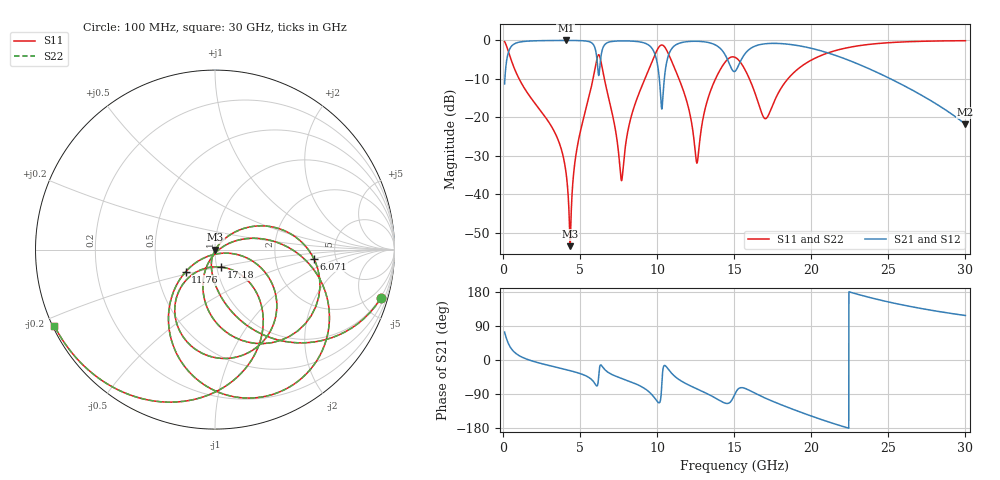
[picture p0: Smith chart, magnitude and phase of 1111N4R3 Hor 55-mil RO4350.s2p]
# GHz S MA R 50
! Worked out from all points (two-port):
!   3201 points, 100 MHz to 30 GHz, reference 50 ohm
!   highest |S21| = -0.02 dB at 4.071 GHz (marker M1); lowest = -21.8 dB at 30 GHz (marker M2)
!   |S21| within 3 dB of the highest: 352.9 MHz to 6.027 GHz (5.674 GHz wide, 178 % of centre); 15.79 GHz to 20.89 GHz (5.094 GHz wide, 27.8 % of centre)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
!   lowest |S11| = -53.5 dB at 4.351 GHz (marker M3), VSWR 1.00, Z = 50.2 - j0.11 ohm
!   |S11| at or under -10 dB: 1.04 GHz to 5.837 GHz (4.797 GHz wide, 140 % of centre); 6.574 GHz to 9.204 GHz (2.63 GHz wide, 33.3 % of centre); 15.98 GHz to 18.48 GHz (2.499 GHz wide, 14.5 % of centre)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
!   |S22| runs from -53.5 to -0.1 dB; largest |S21 - S12| = 0
!   S11 on the Smith chart (normalised r, x): 100 MHz: 0.93, -6.81; 6.071 GHz: 3.40, -0.49; 11.76 GHz: 0.70, -0.18; 17.18 GHz: 1.05, -0.21; 30 GHz: 0.00, -0.23
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0.1  0.9623 -16.4  0.2716 73.6  0.2716 73.6  0.9623 -16.4
1.015688  0.3233 -77.7  0.9456 12.2  0.9456 12.2  0.3233 -77.7
4.071094  0.01998 -110.4  0.9977 -25.2  0.9977 -25.2  0.01998 -110.4
4.351406  0.002103 -31.5  0.9974 -28.1  0.9974 -28.1  0.002103 -31.5
5.089563  0.07556 48.7  0.991 -37.1  0.991 -37.1  0.07556 48.7
6.070656  0.5528 -5.2  0.6197 -68.4  0.6197 -68.4  0.5528 -5.2
6.313594  0.5785 -64.9  0.5312 -13.3  0.5312 -13.3  0.5785 -64.9
6.60325  0.2959 -100.7  0.8825 -25.4  0.8825 -25.4  0.2959 -100.7
7.696469  0.01504 -40.7  0.9842 -48.7  0.9842 -48.7  0.01504 -40.7
9.359656  0.376 4.4  0.8913 -80.3  0.8913 -80.3  0.376 4.4
10.06978  0.7953 -38.6  0.4197 -112.1  0.4197 -112.1  0.7953 -38.6
10.32206  0.8706 -66.0  0.1334 -48.9  0.1334 -48.9  0.8706 -66.0
10.80794  0.6172 -110.3  0.6989 -28.8  0.6989 -28.8  0.6172 -110.3
11.761  0.2044 -142.9  0.9525 -60.1  0.9525 -60.1  0.2044 -142.9
12.59259  0.02547 -72.3  0.9732 -76.5  0.9732 -76.5  0.02547 -72.3
13.52697  0.2384 -18.5  0.9149 -94.8  0.9149 -94.8  0.2384 -18.5
15.05  0.6023 -89.6  0.3961 -89.2  0.3961 -89.2  0.6023 -89.6
15.76013  0.3934 -124.7  0.6943 -75.9  0.6943 -75.9  0.3934 -124.7
17.18038  0.1028 -71.1  0.9099 -103.6  0.9099 -103.6  0.1028 -71.1
20.03956  0.5589 -62.8  0.7854 -148.4  0.7854 -148.4  0.5589 -62.8
25.01978  0.933 -118.7  0.325 153.1  0.325 153.1  0.933 -118.7
30  0.9907 -154.6  0.08114 117.4  0.08114 117.4  0.9907 -154.6
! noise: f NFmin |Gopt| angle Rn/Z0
0.1  0.001232  0.8585  3.231  0.001861
3.417  0.009081  0.4502  23.35  0.002661
6.743  0.07761  0.8425  43.05  0.09057
10.06  0.2897  0.9358  62.07  0.7392
13.39  0.1065  0.7892  80.32  0.06139
16.7  0.1853  0.8464  98.02  0.1114
20.03  0.1328  0.76  112.9  0.0357
23.35  0.1632  0.7819  126.6  0.0328
26.67  0.2567  0.8519  141.2  0.04288
30  0.5599  0.9308  156.9  0.07465
